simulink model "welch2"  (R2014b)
settings: Solver=ode45  StartTime=0.0  StopTime=5  RelTol=1e-3
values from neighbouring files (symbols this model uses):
  w = hanning(N)    [fenster.m]    (also in fourier_transf_puls_3.m = ones(1,N); fourier_transf_puls_4.m = ones(1,N); anti_alias_1.m = sum(hann(nfft).^2)/nfft; anti_alias_2.m = sum(hann(nfft).^2)/nfft)
undefined symbols (not defined in the file or in its folder): fdesignblkfcn, Fs, gcbh, get
libraries: dspstat3 x3, dspspect3 x2, dspsnks4 x2, dspsrcs4 x1, dspsigops x1

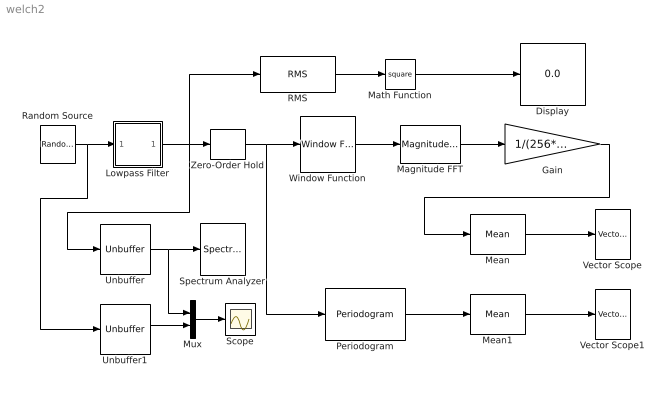
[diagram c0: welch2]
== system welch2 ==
  Display : Display
  Gain : Gain  Gain=1/(256*w*1000)
  Lowpass Filter : Subsystem  DialogController=fdesignblkfcn  InitFcn=fdesignblkfcn(gcbh, {'InitFcn'});
  Magnitude FFT : dspspect3/Magnitude FFT  mag_or_magsq=Magnitude squared  FFTImplementation=Auto  fftLenInherit=off  fftsize=256  WrapInput=off
  Math Function : Math  Operator=square
  Mean : dspstat3/Mean  run=on  reset_popup=None  directionMode=Each column  dimension=1  treatSBRowAsCol=on  roiEnable=off  roiType=Rectangles  roiPortion=Entire ROI  roiOutput=Individual statistics for each ROI  roiFlag=off  outputDataTypeStr=Inherit: Same as accumulator  outputLastDataTypeStr=Inherit: Same as accumulator  outputMin=[]  outputMax=[]  roundingMode=Floor  overflowMode=off
  Mean1 : dspstat3/Mean  run=on  reset_popup=None  directionMode=Each column  dimension=1  treatSBRowAsCol=on  roiEnable=off  roiType=Rectangles  roiPortion=Entire ROI  roiOutput=Individual statistics for each ROI  roiFlag=off  outputDataTypeStr=Inherit: Same as accumulator  outputLastDataTypeStr=Inherit: Same as accumulator  outputMin=[]  outputMax=[]  roundingMode=Floor  overflowMode=off
  Mux : Mux  Inputs=2
  Periodogram : dspspect3/Periodogram  measurement=Power spectral density  wintype=Hamming  Rs=50  beta=5  winsamp=Symmetric  FFTImplementation=Auto  inheritFFT=off  fftsize=256  navg=2  inheritTs=off  Ts=1/1000
  RMS : dspstat3/RMS  run=on  reset_popup=None  InputProcessing=Columns as channels (frame based)  directionMode=Each column  dimension=1  treatSBRowAsCol=on
  Random Source : dspsrcs4/Random Source  SrcType=Gaussian  NormMethod=Ziggurat  CltLength=12  MinVal=0  MaxVal=1  MeanVal=0  VarVal=1  RepMode=Specify seed  rawSeed=78964  IsInherit=off  SampMode=Discrete  SampTime=1/1000  SampFrame=256  DataType=Double  OutComplex=Real
  Scope : Scope
  Spectrum Analyzer : SpectrumAnalyzer
  Unbuffer : Unbuffer  SampleBasedProcessing=Same as frame based
  Unbuffer1 : Unbuffer  SampleBasedProcessing=Same as frame based
  Vector Scope : dspsnks4/Vector Scope  ScopeProperties=on  Domain=Frequency  HorizSpan=1  DisplayProperties=off  AxisGrid=on  Memory=off  FrameNumber=on  AxisLegend=off  AxisZoom=off  OpenScopeAtSimStart=on  OpenScopeImmediately=off  FigPos=get(0,'defaultfigureposition')  AxisProperties=off  XUnits=Hertz  XRange=[-Fs/2...Fs/2]  InheritXIncr=off  XIncr=1/1000  XLabel=Time  XLimit=User-defined  XMin=-500  XMax=500  XStart=0  YUnits=dB  YLabel=Amplitude  LineProperties=off  XAxisParamsVer=6.9
  Vector Scope1 : dspsnks4/Vector Scope  ScopeProperties=on  Domain=Frequency  HorizSpan=1  DisplayProperties=off  AxisGrid=on  Memory=off  FrameNumber=on  AxisLegend=off  AxisZoom=off  OpenScopeAtSimStart=on  OpenScopeImmediately=off  FigPos=[384 509 560 420]  AxisProperties=off  XUnits=Hertz  XRange=[-Fs/2...Fs/2]  InheritXIncr=off  XIncr=1/1000  XLabel=Time  XLimit=User-defined  XMin=-500  XMax=500  XStart=0  YUnits=dB  YLabel=Amplitude  LineProperties=off  XAxisParamsVer=6.9
  Window Function : dspsigops/Window Function  winmode=Apply window to input  wintype=Hamming  sampmode=Continuous  samptime=1  N=64  Rs=50  beta=10  winsamp=Symmetric  UserWindow=hamming  OptParams=off  UserParams={'symmetric'}  RowConvenienceOn=on  dataType=double  isSigned=on  wordLen=16  udDataType=sfix(16)  fracBitsMode=Best precision  numFracBits=15  roundingMode=Floor  overflowMode=off  numSidelobes=4  sidelobeLevel=-30
  Zero-Order Hold : ZeroOrderHold  SampleTime=1/1000
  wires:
  Random Source/1 -> Unbuffer1/1, Lowpass Filter/1(In)
  Window Function/1 -> Magnitude FFT/1
  Magnitude FFT/1 -> Gain/1
  RMS/1 -> Math Function/1
  Lowpass Filter/1(Out) -> Unbuffer/1, RMS/1, Zero-Order Hold/1
  Gain/1 -> Mean/1
  Unbuffer/1 -> Mux/1, Spectrum Analyzer/1
  Mean/1 -> Vector Scope/1
  Math Function/1 -> Display/1
  Periodogram/1 -> Mean1/1
  Zero-Order Hold/1 -> Periodogram/1, Window Function/1
  Mean1/1 -> Vector Scope1/1
  Mux/1 -> Scope/1
  Unbuffer1/1 -> Mux/2

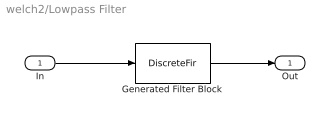
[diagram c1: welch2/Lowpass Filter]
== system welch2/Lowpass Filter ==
  In : Inport
  Generated Filter Block : DiscreteFir  Tag=BlockMethodSubSystem  Coefficients=[0.000837164591190548823 0.000630088428244324227 0.000117016843802876441 -0.00121993975387922442 -0.00332542341352174342 -0.00574692952437155704 -0.00769394282840492674 -0.00829077778658227765 -0.00695524134107234748 -0.00374942375230463915 0.000481574780048023212 0.0043048382956751138 0.00621337352781099316 0.00528242170471527727 0.00168685617863516225 -0.00319545745934425498 -0.00722468309056642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  InputProcessing=Columns as channels (frame based)
  Out : Outport
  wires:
  In/1 -> Generated Filter Block/1
  Generated Filter Block/1 -> Out/1
